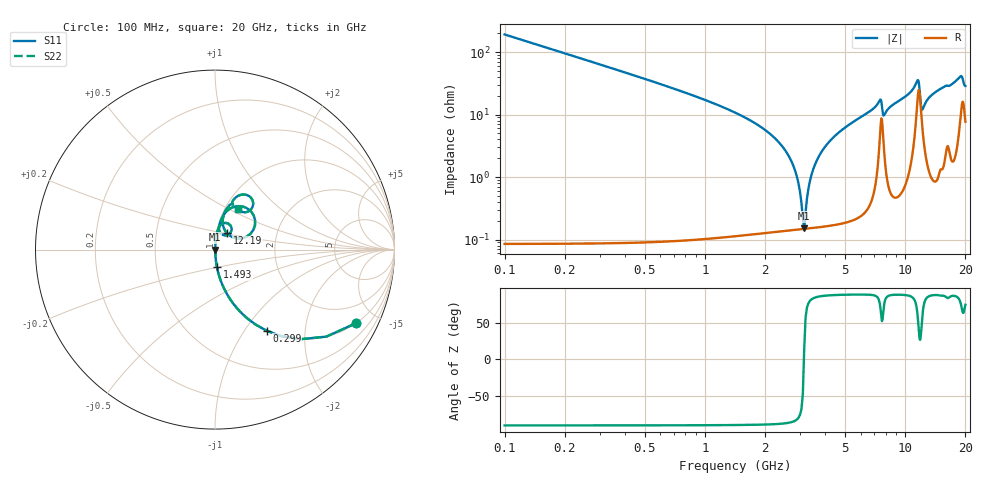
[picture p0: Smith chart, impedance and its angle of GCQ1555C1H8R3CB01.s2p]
!Murata Part Number: GCQ1555C1H8R3CB01
!These Parameters are Measured in Series Mode Connection
!Data Generated on Jan 08, 2026
!  o--ll--o
!Port1  Port2
!  o------o
!Operation Temp=25[degC], DC Bias Voltage=0[V]
!Freq. Start=100[MHz] Stop=20[GHz] 401[Steps]
# Hz S RI R 50
!Freq.(Hz) S11(Real) S11(Imag) S21(Real) S21(Imag) S12(Real) S12(Imag) S22(Real) S22(Imag)
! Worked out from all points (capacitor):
!   401 points, 100 MHz to 20 GHz, reference 50 ohm
!   read as one part in series: C = 8.3 pF near 199.5 MHz
!   lowest |Z| = 152 mohm at 3.135 GHz (marker M1)
!   series resonance near 3.125 GHz, so ESL is about 310 pH
!   S11 on the Smith chart (normalised r, x): 100 MHz: 1.00, -3.83; 299 MHz: 1.00, -1.27; 1.493 GHz: 1.00, -0.20; 12.19 GHz: 1.12, +0.21; 20 GHz: 1.15, +0.55
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1e8  0.7857 -0.4101  0.2143 0.4101  0.2143 0.4101  0.7857 -0.4101
2.99e8  0.2879 -0.4521  0.7121 0.4521  0.7121 0.4521  0.2879 -0.4521
6.4725e8  0.0751 -0.262  0.9249 0.262  0.9249 0.262  0.0751 -0.262
1.493e9  0.0108 -0.098  0.9892 0.098  0.9892 0.098  0.0108 -0.098
2.5875e9  0.00193 -0.0233  0.9981 0.0233  0.9981 0.0233  0.00193 -0.0233
2.83625e9  0.00157 -0.0119  0.9984 0.0119  0.9984 0.0119  0.00157 -0.0119
3.03525e9  0.00147 -0.0036  0.9985 0.0036  0.9985 0.0036  0.00147 -0.0036
3.13475e9  0.00147 0.000377  0.9985 -0.000377  0.9985 -0.000377  0.00147 0.000377
3.43325e9  0.00166 0.0116  0.9983 -0.0116  0.9983 -0.0116  0.00166 0.0116
3.83125e9  0.00224 0.0254  0.9978 -0.0254  0.9978 -0.0254  0.00224 0.0254
4.42825e9  0.00367 0.0443  0.9963 -0.0443  0.9963 -0.0443  0.00367 0.0443
6.7665e9  0.0173 0.1145  0.9827 -0.1145  0.9827 -0.1145  0.0173 0.1145
7.51275e9  0.0735 0.1453  0.9265 -0.1453  0.9265 -0.1453  0.0735 0.1453
7.861e9  0.0328 0.0894  0.9672 -0.0894  0.9672 -0.0894  0.0328 0.0894
1.005e10  0.0436 0.1857  0.9564 -0.1857  0.9564 -0.1857  0.0436 0.1857
1.15425e10  0.2039 0.2087  0.7961 -0.2087  0.7961 -0.2087  0.2039 0.2087
1.189075e10  0.1527 0.0634  0.8473 -0.0634  0.8473 -0.0634  0.1527 0.0634
1.218925e10  0.0675 0.0906  0.9325 -0.0906  0.9325 -0.0906  0.0675 0.0906
1.338325e10  0.0465 0.1856  0.9535 -0.1856  0.9535 -0.1856  0.0465 0.1856
1.67165e10  0.0956 0.2566  0.9044 -0.2566  0.9044 -0.2566  0.0956 0.2566
1.89055e10  0.1911 0.2971  0.8089 -0.2971  0.8089 -0.2971  0.1911 0.2971
2e10  0.1291 0.2241  0.8709 -0.2241  0.8709 -0.2241  0.1291 0.2241
